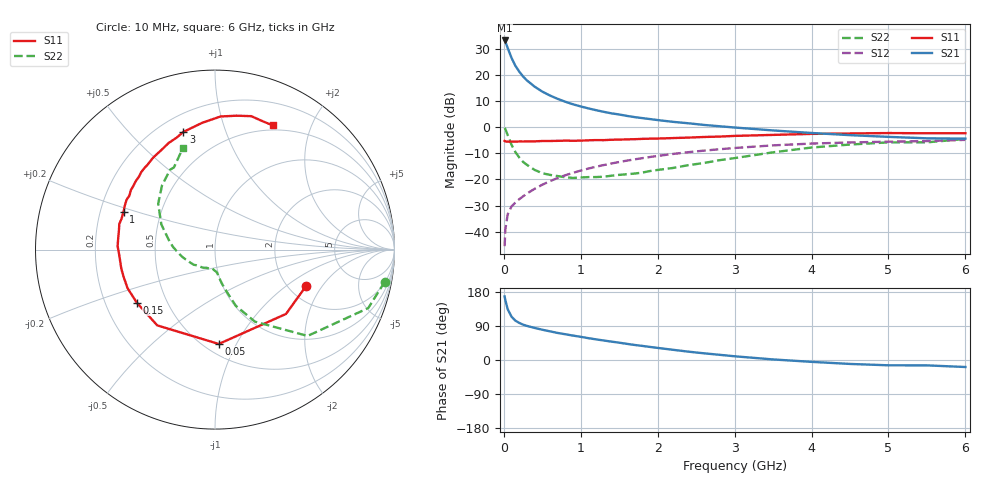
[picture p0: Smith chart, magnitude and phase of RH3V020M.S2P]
! SIEMENS Small Signal Semiconductors
! BFR106
! Si NPN RF Bipolar Junction Transistor in SOT23
! VCE = 3 V  IC = 20 mA
! Common Emitter S-Parameters:  August  1996
# GHz  S  MA  R  50
!  f  S11  S21  S12  S22
! GHz  MAG  ANG  MAG  ANG  MAG  ANG  MAG  ANG
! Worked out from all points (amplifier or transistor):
!   36 points, 10 MHz to 6 GHz, reference 50 ohm
!   highest |S21| = 33.1 dB at 10 MHz (marker M1)
!   |S21| within 3 dB of that: start of sweep to 51.71 MHz
!   unconditionally stable (mu >= 1): 361.5 MHz to 2.278 GHz; 5.357 GHz to end of sweep
!   at 250 MHz: K = 0.90, MSG = 22.9 dB, |S12| = -26.5 dB
!   at 1.4 GHz: K = 1.07, MAG = 7.9 dB, |S12| = -13.9 dB
!   at 6 GHz: K = 1.00, MAG = -0.1 dB, |S12| = -4.9 dB
!   S11 on the Smith chart (normalised r, x): 10 MHz: 2.46, -1.43; 50 MHz: 0.59, -0.85; 150 MHz: 0.34, -0.27; 1 GHz: 0.30, +0.18; 3 GHz: 0.30, +0.72; 6 GHz: 0.44, +1.47
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0.01  0.5462 -22.0  45.36 167.7  0.0053 83.3  0.9631 -10.7
0.02  0.5338 -42.2  42.94 157.6  0.0111 75.6  0.9137 -20.9
0.05  0.5261 -87.7  32.6 134.0  0.0215 59.4  0.7054 -43.0
0.1  0.5308 -127.3  21.04 114.3  0.0305 52.5  0.4591 -61.0
0.15  0.5266 -145.9  14.88 103.9  0.0361 52.9  0.3337 -69.7
0.2  0.5326 -156.2  11.53 97.9  0.0418 55.4  0.2636 -73.1
0.25  0.5313 -163.6  9.295 93.3  0.0474 57.2  0.2162 -76.5
0.3  0.5327 -168.5  7.819 90.0  0.0537 59.9  0.1903 -78.8
0.4  0.5339 -176.3  5.941 84.6  0.0661 62.5  0.1521 -82.1
0.5  0.543 177.9  4.774 79.9  0.0792 64.5  0.1315 -84.5
0.6  0.5432 172.9  4.014 75.6  0.0928 65.1  0.1221 -87.4
0.7  0.5465 168.2  3.468 71.4  0.1065 65.4  0.1159 -91.6
0.8  0.5519 165.1  3.053 67.9  0.1203 65.1  0.11 -95.5
1  0.5516 157.5  2.481 61.1  0.1478 64.0  0.109 -102.3
1.1  0.5594 153.8  2.278 57.6  0.1614 63.3  0.1108 -107.6
1.6  0.5833 139.2  1.638 42.6  0.2288 57.6  0.1257 -130.8
2.2  0.6179 123.8  1.261 26.9  0.3071 49.3  0.1658 -158.1
3  0.6792 105.0  0.983 9.8  0.3992 37.1  0.2558 170.3
3.5  0.7102 95.7  0.864 1.5  0.4479 29.4  0.3301 154.9
4.5  0.7558 80.8  0.702 -10.4  0.5089 14.1  0.4645 129.4
5.5  0.7625 69.1  0.611 -14.2  0.541 4.1  0.5116 116.6
6  0.7635 65.1  0.603 -18.5  0.5706 -3.1  0.5939 107.5
